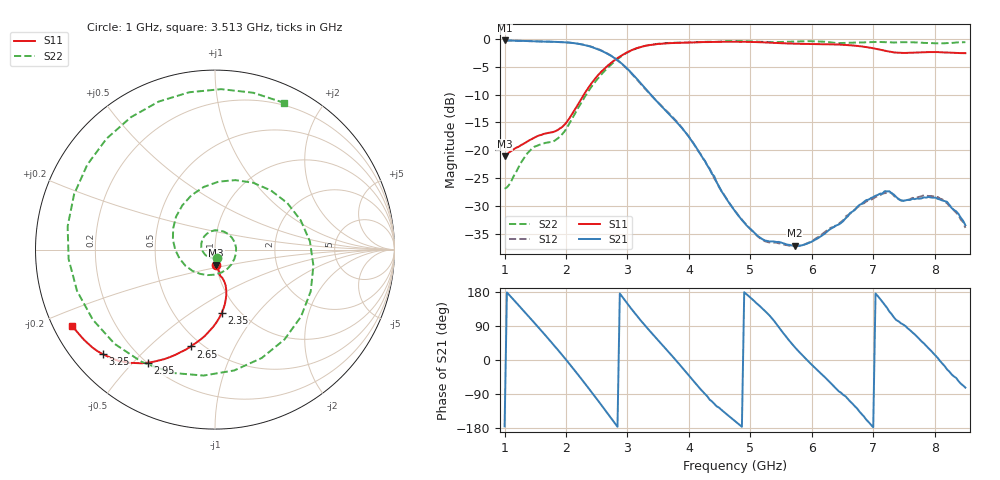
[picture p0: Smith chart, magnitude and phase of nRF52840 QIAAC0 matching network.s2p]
#  HZ  S  RI  R  50.00
! Rohde & Schwarz Vector Network Analyzer
! Rohde-Schwarz,ZNB8-2Port,1311601042101558,2.70
! Created: UTC 10/3/2018, 1:39:30 PM
! freq[Hz]  re:S11  im:S11  re:S21  im:S21  re:S12  im:S12  re:S22  im:S22
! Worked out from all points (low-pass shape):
!   201 points, 1 GHz to 8.5 GHz, reference 50 ohm
!   highest |S21| = -0.29 dB at 1 GHz (marker M1); lowest = -37.1 dB at 5.725 GHz (marker M2)
!   |S21| within 3 dB of the highest: start of sweep to 2.767 GHz
!   lowest |S11| = -21.1 dB at 1 GHz (marker M3), VSWR 1.19, Z = 49.8 - j8.84 ohm
!   |S11| at or under -10 dB: start of sweep to 2.291 GHz
!   |S22| runs from -26.9 to -0.4 dB; largest |S21 - S12| = 0.0082
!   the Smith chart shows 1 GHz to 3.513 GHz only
!   S11 on the Smith chart (normalised r, x): 1 GHz: 1.00, -0.18; 2.35 GHz: 0.83, -0.67; 2.65 GHz: 0.44, -0.68; 2.95 GHz: 0.20, -0.55; 3.25 GHz: 0.09, -0.39; 3.513 GHz: 0.06, -0.25
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1e9  0.00572 -0.0881  -0.9632 -0.0832  -0.9611 -0.084  0.0101 -0.0441
1.5625e9  0.0259 -0.1336  0.1022 0.9425  0.103 0.9429  0.0514 0.0994
2.275e9  0.0556 -0.3009  0.5055 -0.7277  0.5092 -0.7275  -0.2172 0.1831
2.35e9  0.037 -0.3532  0.2826 -0.8181  0.2859 -0.8203  -0.1313 0.3028
2.65e9  -0.1348 -0.5395  -0.5293 -0.5262  -0.536 -0.5267  0.5288 0.0457
2.95e9  -0.3756 -0.6302  -0.5333 0.2042  -0.5272 0.2086  -0.2396 -0.6868
3.25e9  -0.6245 -0.5825  -0.0511 0.3761  -0.0538 0.3717  -0.7114 0.4734
3.5125e9  -0.794 -0.4253  0.1695 0.1993  0.1679 0.2033  0.3833 0.8184
4e9  -0.9259 0.0336  0.0995 -0.0866  0.0987 -0.0886  0.00533 -0.9288
4.3e9  -0.8918 0.2811  -0.00784 -0.0726  -0.00744 -0.0723  -0.9399 0.0464
4.75e9  -0.8169 0.4711  -0.027 -0.00919  -0.0271 -0.00913  0.5024 0.8102
5.275e9  -0.6676 0.6414  -0.00852 0.0128  -0.00815 0.0127  -0.0346 -0.9361
5.725e9  -0.3058 0.8509  0.0116 0.00771  0.0113 0.00791  -0.6771 0.6618
6.025e9  -0.00032 0.8977  0.0148 -0.00441  0.0151 -0.00409  0.4281 0.8483
6.325e9  0.2108 0.8681  0.00887 -0.0179  0.00902 -0.0183  0.9162 -0.1476
6.625e9  0.3514 0.8023  -0.00918 -0.0259  -0.00941 -0.0254  -0.0666 -0.9216
6.925e9  0.5227 0.6538  -0.0347 -0.0101  -0.0339 -0.00978  -0.9249 0.1304
7.2625e9  0.739 0.2119  -0.0263 0.0339  -0.0267 0.0324  0.0749 0.9286
7.6375e9  0.6236 -0.4174  0.0108 0.0352  0.00931 0.0363  0.9285 0.0685
7.975e9  0.338 -0.6815  0.0358 0.0118  0.0369 0.0118  0.0882 -0.9085
8.2375e9  0.0776 -0.7481  0.0281 -0.0165  0.027 -0.0167  -0.9009 -0.1687
8.5e9  -0.2779 -0.6897  0.00627 -0.0204  0.00723 -0.0188  -0.3711 0.8561
